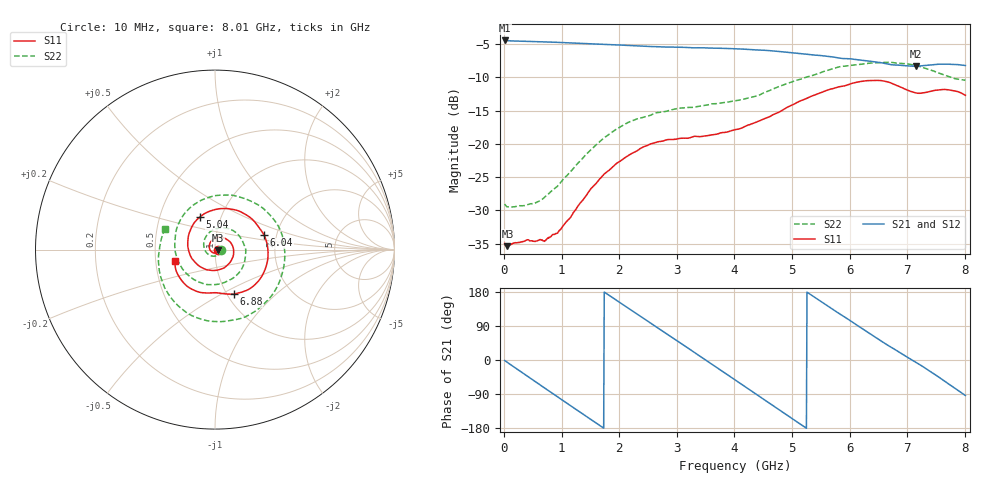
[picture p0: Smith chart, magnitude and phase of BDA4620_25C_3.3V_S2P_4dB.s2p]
!Agilent Technologies,E5071B,MY42404982,A.09.10
!Date: Wed May 06 08:56:49 2026
!Data & Calibration Information:
!Freq	S11:SOLT2(ON)	S21:SOLT2(ON)	S12:SOLT2(ON)	S22:SOLT2(ON)
# Hz S RI R 50
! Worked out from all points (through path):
!   801 points, 10 MHz to 8.01 GHz, reference 50 ohm
!   highest |S21| = -4.45 dB at 10 MHz (marker M1); lowest = -8.3 dB at 7.15 GHz (marker M2)
!   group delay of S21, straight-line fit = 282 ps
!   lowest |S11| = -35.4 dB at 60 MHz (marker M3), VSWR 1.03, Z = 51.7 - j0.181 ohm
!   |S11| at or under -10 dB: start of sweep to end of sweep
!   |S22| runs from -29.5 to -7.7 dB; largest |S21 - S12| = 0.0024
!   S11 on the Smith chart (normalised r, x): 10 MHz: 1.04, -0.00; 5.04 GHz: 0.79, +0.30; 6.04 GHz: 1.72, +0.30; 6.88 GHz: 1.07, -0.57; 8.01 GHz: 0.63, -0.08
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1e7  0.0178 -0.00112  0.5991 -0.0128  0.5998 -0.0132  0.0352 -0.00278
6e7  0.0169 -0.00175  0.5926 -0.0685  0.5941 -0.0693  0.0331 -0.00613
3.7e8  0.0147 -0.0115  0.4588 -0.3716  0.4588 -0.3724  0.0187 -0.029
7.3e8  -0.00166 -0.019  0.1361 -0.5677  0.1359 -0.5686  -0.0199 -0.0355
1.03e9  -0.0223 -0.00979  -0.1751 -0.5505  -0.1754 -0.551  -0.0537 -0.00856
1.35e9  -0.032 0.0186  -0.4415 -0.361  -0.4419 -0.3613  -0.061 0.0466
1.65e9  -0.0173 0.0508  -0.5561 -0.0825  -0.5569 -0.0826  -0.027 0.0992
1.94e9  0.0178 0.0681  -0.5172 0.2011  -0.5182 0.2016  0.0395 0.122
2.32e9  0.0723 0.0525  -0.2714 0.473  -0.2722 0.4734  0.1321 0.0801
2.68e9  0.1039 -0.000919  0.0599 0.534  0.0605 0.5342  0.1715 -0.0152
3e9  0.091 -0.0595  0.3341 0.4158  0.3349 0.4155  0.1466 -0.1118
3.39e9  0.0351 -0.1078  0.5174 0.1057  0.5178 0.1048  0.0373 -0.188
4.01e9  -0.091 -0.0894  0.3173 -0.4102  0.317 -0.411  -0.1826 -0.1054
4.5e9  -0.1518 0.0215  -0.1136 -0.4934  -0.1142 -0.4939  -0.2163 0.1064
5.04e9  -0.0856 0.18  -0.4495 -0.1758  -0.4499 -0.1752  -0.0185 0.2954
5.35e9  0.0261 0.2281  -0.4602 0.0815  -0.46 0.0821  0.1533 0.2876
6.04e9  0.2737 0.0794  -0.0808 0.4268  -0.0803 0.4271  0.3891 -0.0291
6.68e9  0.1903 -0.2202  0.3157 0.2402  0.3172 0.2404  0.1804 -0.3689
6.88e9  0.1034 -0.2472  0.3688 0.1255  0.3702 0.1251  0.0487 -0.4005
7.15e9  0.0151 -0.2411  0.3813 -0.0414  0.3821 -0.0421  -0.1357 -0.3645
7.57e9  -0.1227 -0.2236  0.2683 -0.2933  0.2686 -0.2941  -0.3025 -0.1516
8.01e9  -0.2236 -0.0618  -0.0241 -0.3876  -0.0247 -0.3886  -0.2779 0.1144
